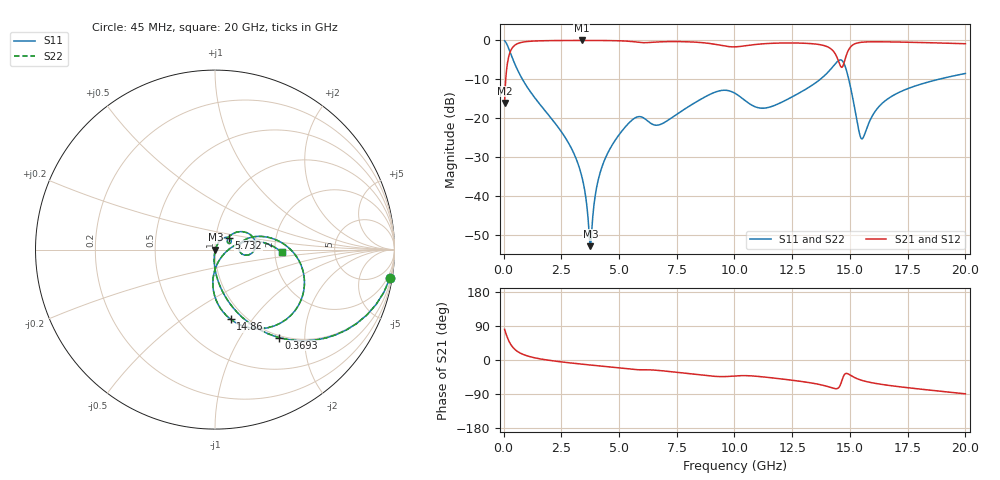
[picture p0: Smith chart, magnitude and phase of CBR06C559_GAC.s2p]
! S-parameter model data by Modelithics Inc.  support@modelithics.com 813-866-6335  Tampa FL USA
! S-Parameter data specifications:
! Substrate: 20-mil Rogers 4350B, substrate thickness, H=0.508mm, Dielectric constant, Er=3.75
! PCB Mounting Pad Footprint: Pad width, PadW=0.85mm , Pad length, PadL=0.64mm , Pad gap, PadG (edge-to-edge)=0.62mm , Reference planes=1.9mm apart
#  GHz  S  MA  R 50
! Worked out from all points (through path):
!   801 points, 45 MHz to 20 GHz, reference 50 ohm
!   highest |S21| = -0.02 dB at 3.387 GHz (marker M1); lowest = -16.1 dB at 45 MHz (marker M2)
!   group delay of S21, straight-line fit = 13.6 ps
!   lowest |S11| = -53.0 dB at 3.762 GHz (marker M3), VSWR 1.00, Z = 50.2 - j0.0404 ohm
!   |S11| at or under -10 dB: 814.9 MHz to 13.72 GHz (12.9 GHz wide, 178 % of centre); 14.95 GHz to 18.86 GHz (3.909 GHz wide, 23.1 % of centre)
!   |S22| runs from -53.0 to -0.1 dB; largest |S21 - S12| = 0
!   S11 on the Smith chart (normalised r, x): 45 MHz: 1, -12; 369.3 MHz: 0.97, -1.50; 5.732 GHz: 1.16, +0.15; 14.86 GHz: 0.86, -0.79; 20 GHz: 2.20, -0.08
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0.045  0.9876 -9.2  0.1567 80.8  0.1567 80.8  0.9876 -9.2
0.194662  0.8237 -35.2  0.5665 54.8  0.5665 54.8  0.8237 -35.2
0.369269  0.6056 -54.0  0.795 36.0  0.795 36.0  0.6056 -54.0
1.067694  0.2393 -79.7  0.9698 10.1  0.9698 10.1  0.2393 -79.7
2.738925  0.05203 -95.0  0.997 -6.7  0.997 -6.7  0.05203 -95.0
3.387462  0.01773 -94.9  0.9978 -10.9  0.9978 -10.9  0.01773 -94.9
3.761619  0.002241 -10.3  0.9976 -13.3  0.9976 -13.3  0.002241 -10.3
4.036  0.01308 63.0  0.997 -15.0  0.997 -15.0  0.01308 63.0
4.360269  0.02816 65.5  0.9957 -17.0  0.9957 -17.0  0.02816 65.5
5.732175  0.1018 39.7  0.9526 -25.4  0.9526 -25.4  0.1018 39.7
6.704981  0.08132 31.8  0.9557 -27.5  0.9557 -27.5  0.08132 31.8
9.074637  0.2105 24.3  0.8987 -42.8  0.8987 -42.8  0.2105 24.3
10.0225  0.2084 -4.8  0.8257 -42.1  0.8257 -42.1  0.2084 -4.8
11.31958  0.1344 4.8  0.9075 -45.1  0.9075 -45.1  0.1344 4.8
13.36496  0.2649 16.1  0.9061 -61.0  0.9061 -61.0  0.2649 16.1
14.08833  0.4005 2.7  0.8099 -71.0  0.8099 -71.0  0.4005 2.7
14.46249  0.5356 -21.5  0.5836 -75.1  0.5836 -75.1  0.5356 -21.5
14.66204  0.5483 -48.4  0.4515 -52.4  0.4515 -52.4  0.5483 -48.4
14.86159  0.3985 -77.3  0.6664 -35.5  0.6664 -35.5  0.3985 -77.3
15.51013  0.05396 -41.4  0.9464 -53.6  0.9464 -53.6  0.05396 -41.4
16.68248  0.1804 14.5  0.9566 -67.0  0.9566 -67.0  0.1804 14.5
20  0.3751 -2.5  0.9052 -89.3  0.9052 -89.3  0.3751 -2.5
